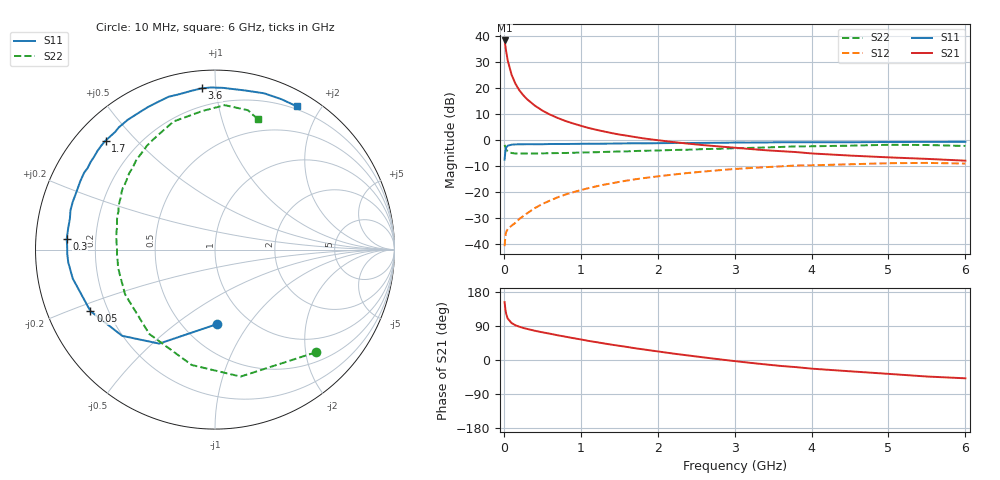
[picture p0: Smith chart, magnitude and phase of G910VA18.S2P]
! SIEMENS Small Signal Semiconductors
! BFG235
! Si NPN RF Bipolar Junction Transistor in SOT223
! VCE = 10 V  IC = 180 mA
! Common Emitter S-Parameters:  July  1994
# GHz  S  MA  R  50
!  f  S11  S21  S12  S22
! GHz  MAG  ANG  MAG  ANG  MAG  ANG  MAG  ANG
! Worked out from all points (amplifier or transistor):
!   40 points, 10 MHz to 6 GHz, reference 50 ohm
!   highest |S21| = 38.4 dB at 10 MHz (marker M1)
!   |S21| within 3 dB of that: start of sweep to 24.6 MHz
!   unconditionally stable (mu >= 1): 450.2 MHz to 1.5 GHz
!   at 200 MHz: K = 0.81, MSG = 24.9 dB, |S12| = -30.5 dB
!   at 1.5 GHz: K = 1.00, MSG = 9.1 dB, |S12| = -16.2 dB
!   at 6 GHz: K = 0.89, MSG = 0.6 dB, |S12| = -9.1 dB
!   S11 on the Smith chart (normalised r, x): 10 MHz: 0.72, -0.72; 50 MHz: 0.13, -0.23; 300 MHz: 0.09, +0.03; 1.7 GHz: 0.09, +0.41; 3.6 GHz: 0.10, +0.92; 6 GHz: 0.17, +1.71
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0.01  0.416 -88.8  83.24 152.7  0.0089 62.2  0.802 -45.5
0.02  0.6091 -120.7  65.92 133.8  0.0139 48.0  0.7217 -78.6
0.03  0.7059 -137.1  51.67 122.1  0.0166 40.9  0.6559 -101.4
0.05  0.774 -153.7  34.45 109.5  0.0191 34.2  0.5958 -127.9
0.1  0.8088 -168.5  18.22 97.6  0.0221 37.0  0.5596 -153.5
0.15  0.8206 -175.0  12.23 91.7  0.0251 44.0  0.5485 -164.0
0.2  0.8236 -178.3  9.152 88.0  0.0297 49.1  0.5491 -169.7
0.25  0.824 178.5  7.372 84.7  0.0337 53.0  0.546 -173.5
0.3  0.8284 176.0  6.151 82.2  0.0381 55.8  0.5466 -176.8
0.4  0.8266 171.5  4.627 77.3  0.0481 58.7  0.5461 178.9
0.5  0.8266 168.0  3.695 73.1  0.0579 60.1  0.5507 175.5
0.6  0.8346 164.7  3.083 69.4  0.0676 60.6  0.5546 172.4
0.8  0.8357 158.4  2.326 61.6  0.0883 59.5  0.5596 167.1
1.1  0.8456 149.6  1.705 50.4  0.1174 55.8  0.5762 160.2
1.4  0.8495 142.4  1.358 40.5  0.1453 51.1  0.5931 154.2
1.7  0.8604 135.1  1.142 31.2  0.1733 45.9  0.6107 148.6
2.2  0.8713 124.0  0.911 17.0  0.2146 36.7  0.64 138.4
3.2  0.8884 102.8  0.669 -7.4  0.2867 17.4  0.7018 119.8
3.6  0.9014 94.7  0.607 -15.7  0.3094 9.1  0.7316 111.5
4.5  0.9024 79.2  0.499 -29.8  0.3389 -7.2  0.7755 95.2
5.5  0.916 66.1  0.431 -43.6  0.3602 -25.4  0.798 76.7
6  0.9191 60.2  0.398 -48.3  0.35 -32.3  0.7649 71.9
